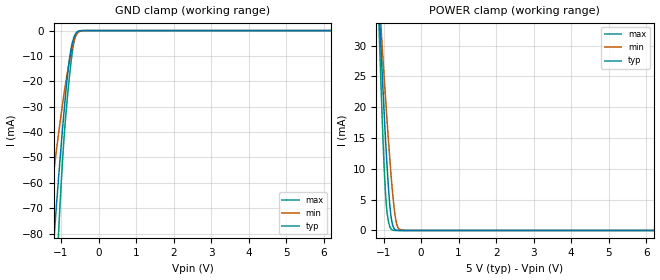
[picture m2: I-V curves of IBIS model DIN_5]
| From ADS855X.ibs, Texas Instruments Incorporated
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|   INPUT 5.0V Model
[Model]   DIN_5
Model_type   Input
| Signals   CS/FS, RD, CONVST_C, CONVST_B, CONVST_A, STBY, RANGE/XCLK,
|   RESET, WORD/BYTE, PAR/SER, HW/SW,REFEN/WR
Vinl = -300.000mV   |min, BGND -0.3V
Vinh = 5.8V   |max. BVDD +0.3V
| C_comp   obtained at 25MHz
| variable   typ   min   max
C_comp   3.408pF   2.584pF   4.227pF
[Temperature Range]   40.0   125.0   -40.0
[Voltage range]   5.0V   4.50V   5.50V
[power clamp reference] 5.0V   4.50V   5.50V
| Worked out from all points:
|   GND clamp passes 1 mA (typ) near -0.60 V on its own axis
|   POWER clamp passes 1 mA (typ) near -0.76 V on its own axis
[GND Clamp]
|   Voltage   I(typ)   I(min)   I(max)
-5V       -965.7mA   -668.8mA   -1.352A
-1.402V   -126.5mA   -82.34mA   -183.3mA
-1.312V   -107.4mA   -70.57mA   -154.8mA
-1.166V   -77.55mA   -52.34mA   -109.4mA
-1.094V   -63.6mA    -43.91mA   -88.07mA
-1.053V   -55.75mA   -39.19mA   -76.11mA
-968.8mV  -40.35mA   -29.96mA   -53.42mA
-914.4mV  -31.04mA   -24.37mA   -41.2mA
-771.9mV  -10.89mA   -11.62mA   -17.61mA
-651.9mV  -2.469mA   -4.02mA    -4.15mA
-522.5mV  -179.9uA   -465.9uA   -188.1uA
9.998V    0A         0A         0A
[POWER Clamp]
|   Voltage   I(typ)   I(min)   I(max)
-5V       320.7mA    274.7mA    381.2mA
-1.117V   36.27mA    38.08mA    32.47mA
-1.055V   28.03mA    31.85mA    21.43mA
-1.001V   21.14mA    26.56mA    12.71mA
-953.8mV  15.6mA     22.17mA    6.678mA
-914.4mV  11.3mA     18.6mA     3.371mA
-869.4mV  6.963mA    14.67mA    1.459mA
-828.1mV  3.801mA    11.25mA    561.2uA
-770mV    1.186mA    6.872mA    84.49uA
-657.5mV  45.3uA     1.24mA     2.004uA
-485mV    108nA      12.27uA    43.95nA
9.998V    0A         0A         0A
